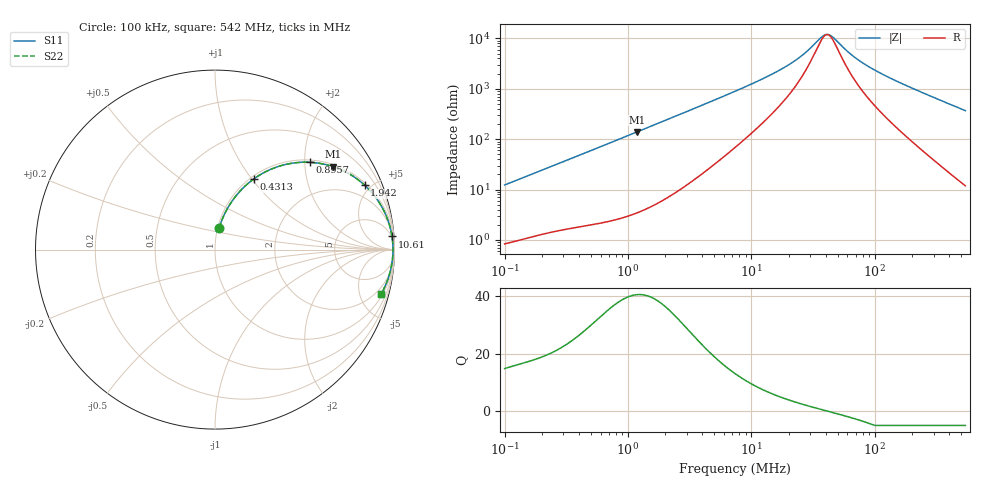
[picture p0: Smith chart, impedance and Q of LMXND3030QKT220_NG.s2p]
! LMXND3030QKT220_NG  S-PARAMETER MODEL  ( General Type )
! Model Generated by TAIYO YUDEN Corporation (http://www.ty-top.com)
! Version 1.0
! TAIYO YUDEN Control No. 191023NI43SB-FBB
! Copyright(c) 2019 TAIYO YUDEN CO.,LTD. All Rights Reserved.
! Product Description (link to TY-COMPAS)
! https://ds.yuden.co.jp/TYCOMPAS/or/detail?pn=LMXND3030QKT220MNG&u=M
! Products Name : Inductors
! Characteristics :
!  Inductance : 22 uH , SRF(min) : 20 MHz , DC Resistance(max) : 0.624 Ohm
!  Rated Current : Saturation :470 mA , Temp Rise : 470 mA
!  Case Size : 3.0 x 3.0 / 0.118 x 0.118 [mm/inch] , Thickness : 1.5 / 0.059 [mm/inch]
!  (Conditions: Temperature = 25 degC , DC Bias Current/Voltage = 0A / 0V)
! External Node Assignments :
!  1  o---GGG---o  2
! GND o---------o GND
! Frequency Range : 0.1MHz  -  542.002916MHz  [ 402 STEP ]
# MHz S RI R 50
! Freq[MHz].  S11 Real  S11 Imag  S21 Real  S21 Imag  S12 Real  S12 Imag  S22 Real  S22 Imag
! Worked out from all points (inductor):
!   401 points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, 100 kHz to 542 MHz, reference 50 ohm
!   read as one part in series: L = 19.5 uH near 104.4 kHz
!   highest Q = 40.5 at 1.184 MHz (marker M1), where L = 18.8 uH
!   self-resonance near 41.1 MHz
!   S11 on the Smith chart (normalised r, x): 100 kHz: 1.02, +0.25; 431.3 kHz: 1.04, +1.02; 895.7 kHz: 1.05, +2.11; 1.942 MHz: 1.12, +4.58; 10.61 MHz: 4, +26; 542 MHz: 1.24, -7.38
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0.1  0.0229 0.1195  0.9771 -0.1195  0.9771 -0.1195  0.0229 0.1195
0.231241  0.083 0.252  0.917 -0.252  0.917 -0.252  0.083 0.252
0.422129  0.2099 0.3892  0.7901 -0.3892  0.7901 -0.3892  0.2099 0.3892
0.431301  0.2165 0.3941  0.7835 -0.3941  0.7835 -0.3941  0.2165 0.3941
0.648852  0.3742 0.4695  0.6258 -0.4695  0.6258 -0.4695  0.3742 0.4695
0.895716  0.5272 0.4865  0.4728 -0.4865  0.4728 -0.4865  0.5272 0.4865
1.184474  0.6576 0.4623  0.3424 -0.4623  0.3424 -0.4623  0.6576 0.4623
1.78193  0.8092 0.38  0.1908 -0.38  0.1908 -0.38  0.8092 0.38
1.941917  0.8334 0.3593  0.1666 -0.3593  0.1666 -0.3593  0.8334 0.3593
3.395789  0.934 0.2299  0.066 -0.2299  0.066 -0.2299  0.934 0.2299
7.362085  0.9795 0.1085  0.0205 -0.1085  0.0205 -0.1085  0.9795 0.1085
10.60952  0.9862 0.0731  0.0138 -0.0731  0.0138 -0.0731  0.9862 0.0731
20.21836  0.9907 0.0313  0.00928 -0.0313  0.00928 -0.0313  0.9907 0.0313
25.61127  0.9913 0.02  0.00868 -0.02  0.00868 -0.02  0.9913 0.02
31.0775  0.9916 0.0115  0.00841 -0.0115  0.00841 -0.0115  0.9916 0.0115
37.7104  0.9917 0.00352  0.00828 -0.00352  0.00828 -0.00352  0.9917 0.00352
40.22223  0.9917 0.000892  0.00827 -0.000892  0.00827 -0.000892  0.9917 0.000892
42.90137  0.9917 -0.00173  0.00827 0.00173  0.00827 0.00173  0.9917 -0.00173
73.42539  0.9911 -0.0249  0.00889 0.0249  0.00889 0.0249  0.9911 -0.0249
131.1872  0.9883 -0.0583  0.0117 0.0583  0.0117 0.0583  0.9883 -0.0583
278.3662  0.9737 -0.1321  0.0263 0.1321  0.0263 0.1321  0.9737 -0.1321
542.0029  0.9247 -0.2483  0.0753 0.2483  0.0753 0.2483  0.9247 -0.2483
